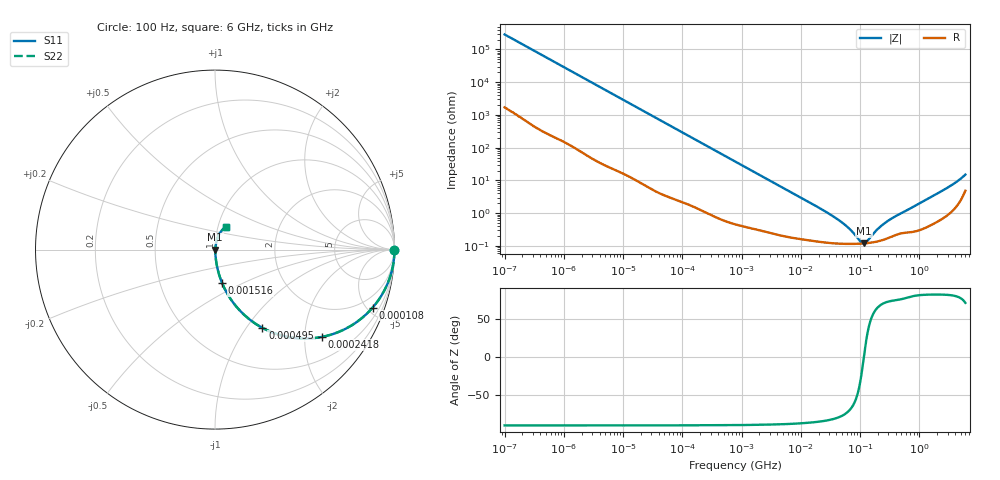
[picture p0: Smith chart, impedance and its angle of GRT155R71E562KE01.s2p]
!Murata Part Number: GRT155R71E562KE01
!These Parameters are Measured in Series Mode Connection
!Data Generated on Jun 19, 2026
!  o--ll--o
!Port1  Port2
!  o------o
!Operation Temp=25[degC], DC Bias Voltage=0[V]
!Freq. Start=100[Hz] Stop=6[GHz] 401[Steps]
# Hz S RI R 50
!Freq.(Hz) S11(Real) S11(Imag) S21(Real) S21(Imag) S12(Real) S12(Imag) S22(Real) S22(Imag)
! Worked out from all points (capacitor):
!   401 points, 100 Hz to 6 GHz, reference 50 ohm
!   read as one part in series: C = 5.56 nF near 109 Hz
!   lowest |Z| = 120 mohm at 116.7 MHz (marker M1)
!   series resonance near 115.9 MHz, so ESL is about 340 pH
!   S11 on the Smith chart (normalised r, x): 100 Hz: open; 108 kHz: 1.04, -5.42; 241.8 kHz: 1.02, -2.43; 495 kHz: 1.01, -1.19; 1.516 MHz: 1.01, -0.39; 6 GHz: 1.10, +0.29
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100  1 -0.00035  2.2e-06 0.00035  2.2e-06 0.00035  1 -0.00035
2008  0.9999 -0.00695  8.33e-05 0.00695  8.33e-05 0.00695  0.9999 -0.00695
12592  0.9979 -0.0432  0.00212 0.0432  0.00212 0.0432  0.9979 -0.0432
40335  0.9805 -0.1355  0.0195 0.1355  0.0195 0.1355  0.9805 -0.1355
108014  0.8783 -0.3232  0.1217 0.3232  0.1217 0.3232  0.8783 -0.3232
161617  0.7653 -0.4197  0.2347 0.4197  0.2347 0.4197  0.7653 -0.4197
241822  0.5956 -0.4864  0.4044 0.4864  0.4044 0.4864  0.5956 -0.4864
345986  0.4209 -0.4891  0.5791 0.4891  0.5791 0.4891  0.4209 -0.4891
495019  0.2641 -0.4358  0.7359 0.4358  0.7359 0.4358  0.2641 -0.4358
774597  0.13 -0.3303  0.87 0.3303  0.87 0.3303  0.13 -0.3303
1516199  0.0399 -0.1872  0.9601 0.1872  0.9601 0.1872  0.0399 -0.1872
4060267  0.00754 -0.0729  0.9925 0.0729  0.9925 0.0729  0.00754 -0.0729
1.555665e7  0.0018 -0.0191  0.9982 0.0191  0.9982 0.0191  0.0018 -0.0191
4.764863e7  0.0012 -0.00536  0.9988 0.00536  0.9988 0.00536  0.0012 -0.00536
6.817316e7  0.00116 -0.00295  0.9988 0.00295  0.9988 0.00295  0.00116 -0.00295
1.020051e8  0.00118 -0.000679  0.9988 0.000679  0.9988 0.000679  0.00118 -0.000679
1.166697e8  0.00119 3.51e-05  0.9988 -3.51e-05  0.9988 -3.51e-05  0.00119 3.51e-05
1.334425e8  0.00122 0.000749  0.9988 -0.000749  0.9988 -0.000749  0.00122 0.000749
2.088084e8  0.00142 0.00327  0.9986 -0.00327  0.9986 -0.00327  0.00142 0.00327
3.124326e8  0.00183 0.00595  0.9982 -0.00595  0.9982 -0.00595  0.00183 0.00595
2.802721e9  0.0109 0.0544  0.9891 -0.0544  0.9891 -0.0544  0.0109 0.0544
6e9  0.064 0.1278  0.936 -0.1278  0.936 -0.1278  0.064 0.1278
